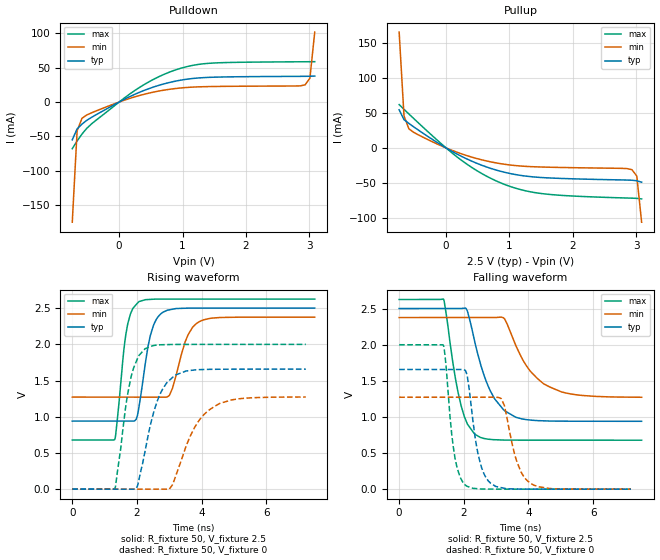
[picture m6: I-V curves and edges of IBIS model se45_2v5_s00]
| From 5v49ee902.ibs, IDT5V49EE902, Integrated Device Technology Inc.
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[Model]   se45_2v5_s00
Model_type   Output
Polarity   Non-Inverting
|   typ   min   max
C_comp   2pF   1.5pF   2.5pF
Vmeas = 1.25V
Rref = 50
Cref = 0
Vref = 1.25V
|   typ   min   max
[Voltage range]   2.5V   2.375V   2.625V
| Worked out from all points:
|   slope of the pulldown table from 0 to 0.375 V, typ, clamps not added: 23.2 ohm
|   slope of the pullup table from 0 to 0.375 V, typ, clamps not added: 21 ohm
|   rising waveform, R_fixture 50, V_fixture 2.5: 20-80 % time 355ps typ, 450ps min, 276ps max; typ from 0.939 V to 2.5 V
|   falling waveform, R_fixture 50, V_fixture 2.5: 20-80 % time 687ps typ, 919ps min, 460ps max; typ from 2.5 V to 0.939 V
|   rising waveform, R_fixture 50, V_fixture 0: 20-80 % time 568ps typ, 790ps min, 399ps max; typ from 0 V to 1.66 V
|   falling waveform, R_fixture 50, V_fixture 0: 20-80 % time 345ps typ, 432ps min, 272ps max; typ from 1.66 V to 0 V
[Pulldown]
|Voltage   I (typ)   I (min)   I (max)
|Note, modeling breaks down at 250mA and above.  This is well beyond the functional   |
|operating range of the device.  Should this scenario occur, catastrophic failure and   |
|possible damage to the device and/or board is of higher concern than the I-V curve   |
|behavior.  The IBIS checker will flag currents in excess of 10A with warnings.  Lines   |
|with currents in excess of 0.35 A have been commented out.  The points still remain|
|available to the user if the user desires to use them.   |
|-2.50000e+00   -4.54709e+01   -3.63694e+01   -6.07959e+01
|-2.42347e+00   -4.32502e+01   -3.46594e+01   -5.77053e+01
|-2.34694e+00   -4.10314e+01   -3.29511e+01   -5.46170e+01
|-2.27041e+00   -3.88148e+01   -3.12446e+01   -5.15313e+01
|-2.19388e+00   -3.66007e+01   -2.95401e+01   -4.84486e+01
|-2.11735e+00   -3.43893e+01   -2.78380e+01   -4.53691e+01
|-2.04082e+00   -3.21809e+01   -2.61384e+01   -4.22934e+01
|-1.96429e+00   -2.99761e+01   -2.44418e+01   -3.92219e+01
|-1.88776e+00   -2.77753e+01   -2.27484e+01   -3.61555e+01
|-1.81122e+00   -2.55791e+01   -2.10589e+01   -3.30948e+01
|-1.73469e+00   -2.33884e+01   -1.93737e+01   -3.00411e+01
|-1.65816e+00   -2.12042e+01   -1.76937e+01   -2.69958e+01
|-1.58163e+00   -1.90279e+01   -1.60198e+01   -2.39607e+01
|-1.50510e+00   -1.68611e+01   -1.43533e+01   -2.09385e+01
|-1.42857e+00   -1.47065e+01   -1.26960e+01   -1.79331e+01
|-1.35204e+00   -1.25675e+01   -1.10500e+01   -1.49501e+01
|-1.27551e+00   -1.04495e+01   -9.41889e+00   -1.19989e+01
|-1.19898e+00   -8.36102e+00   -7.80755e+00   -9.09553e+00
|-1.12245e+00   -6.31683e+00   -6.22400e+00   -6.27207e+00
|-1.04592e+00   -4.34540e+00   -4.68188e+00   -3.60463e+00
|-9.69388e-01   -2.51112e+00   -3.20700e+00   -1.33260e+00
|-8.92857e-01   -9.89892e-01   -1.85502e+00   -2.01598e-01
|-8.16327e-01   -1.92135e-01   -7.61074e-01   -8.24374e-02
-739.8mV  -54.82mA   -174.4mA   -67.73mA
-663.3mV  -39mA      -41.68mA   -56.5mA
-586.7mV  -31.96mA   -23.62mA   -46.47mA
-433.7mV  -22.15mA   -15.6mA    -31.55mA
255.1mV   11.54mA    7.746mA    17.23mA
637.8mV   24.55mA    16.14mA    37.26mA
943.9mV   31.29mA    20.16mA    48.22mA
1.173V    34.28mA    21.72mA    53.44mA
1.48V     36mA       22.52mA    56.56mA
2.934V    37.31mA    24.91mA    58.47mA
3.01V     37.39mA    34.58mA    58.51mA
3.087V    37.69mA    101.5mA    58.57mA
| 3.16327e+00   3.94370e-02   3.90716e-01   5.87161e-02
| 3.23980e+00   5.34569e-02   9.26332e-01   5.92247e-02
| 3.31633e+00   1.87777e-01   1.58664e+00   6.05142e-02
| 3.39286e+00   7.03900e-01   2.30650e+00   6.31621e-02
| 3.46939e+00   1.49296e+00   3.05902e+00   8.17834e-02
| 3.54592e+00   2.39302e+00   3.83167e+00   3.62573e-01
| 3.62245e+00   3.34512e+00   4.61786e+00   1.23067e+00
| 3.69898e+00   4.32630e+00   5.41369e+00   2.35283e+00
| 3.77551e+00   5.32579e+00   6.21672e+00   3.56536e+00
| 3.85204e+00   6.33779e+00   7.02533e+00   4.82080e+00
| 3.92857e+00   7.35883e+00   7.83838e+00   6.10084e+00
| 4.00510e+00   8.38670e+00   8.65504e+00   7.39669e+00
| 4.08163e+00   9.41993e+00   9.47469e+00   8.70352e+00
| 4.15816e+00   1.04574e+01   1.02969e+01   1.00184e+01
| 4.23469e+00   1.14984e+01   1.11212e+01   1.13394e+01
| 4.31122e+00   1.25424e+01   1.19474e+01   1.26653e+01
| 4.38776e+00   1.35888e+01   1.27751e+01   1.39952e+01
| 4.46429e+00   1.46373e+01   1.36044e+01   1.53282e+01
| 4.54082e+00   1.56877e+01   1.44348e+01   1.66640e+01
| 4.61735e+00   1.67397e+01   1.52665e+01   1.80021e+01
| 4.69388e+00   1.77932e+01   1.60991e+01   1.93422e+01
| 4.77041e+00   1.88479e+01   1.69326e+01   2.06841e+01
| 4.84694e+00   1.99037e+01   1.77670e+01   2.20275e+01
| 4.92347e+00   2.09606e+01   1.86021e+01   2.33723e+01
| 5.00000e+00   2.20184e+01   1.94379e+01   2.47183e+01
[Pullup]
|Voltage   I (typ)   I (min)   I (max)
|Note, modeling breaks down at 250mA and above.  This is well beyond the functional   |
|operating range of the device.  Should this scenario occur, catastrophic failure and   |
|possible damage to the device and/or board is of higher concern than the I-V curve   |
|behavior.  The IBIS checker will flag currents in excess of 10A with warnings.  Lines   |
|with currents in excess of 0.35 A have been commented out.  The points still remain|
|available to the user if the user desires to use them.   |
|-2.50000e+00   2.19765e+01   1.80472e+01   2.68517e+01
|-2.42347e+00   2.09191e+01   1.72127e+01   2.55048e+01
|-2.34694e+00   1.98626e+01   1.63791e+01   2.41589e+01
|-2.27041e+00   1.88071e+01   1.55463e+01   2.28141e+01
|-2.19388e+00   1.77528e+01   1.47145e+01   2.14705e+01
|-2.11735e+00   1.66997e+01   1.38838e+01   2.01283e+01
|-2.04082e+00   1.56480e+01   1.30543e+01   1.87877e+01
|-1.96429e+00   1.45980e+01   1.22261e+01   1.74489e+01
|-1.88776e+00   1.35497e+01   1.13995e+01   1.61122e+01
|-1.81122e+00   1.25036e+01   1.05747e+01   1.47780e+01
|-1.73469e+00   1.14600e+01   9.75186e+00   1.34466e+01
|-1.65816e+00   1.04193e+01   8.93142e+00   1.21187e+01
|-1.58163e+00   9.38215e+00   8.11380e+00   1.07950e+01
|-1.50510e+00   8.34928e+00   7.29955e+00   9.47668e+00
|-1.42857e+00   7.32178e+00   6.48942e+00   8.16516e+00
|-1.35204e+00   6.30119e+00   5.68442e+00   6.86272e+00
|-1.27551e+00   5.28973e+00   4.88602e+00   5.57292e+00
|-1.19898e+00   4.29091e+00   4.09630e+00   4.30185e+00
|-1.12245e+00   3.31066e+00   3.31857e+00   3.06117e+00
|-1.04592e+00   2.36002e+00   2.55827e+00   1.87712e+00
|-9.69388e-01   1.46263e+00   1.82537e+00   8.26238e-01
|-8.92857e-01   6.79721e-01   1.14025e+00   1.77022e-01
|-8.16327e-01   1.78304e-01   5.50947e-01   7.20287e-02
-739.8mV  54.64mA    166.3mA    62.19mA
-663.3mV  40.61mA    45.96mA    55.4mA
-586.7mV  35.13mA    27.42mA    48.78mA
-204.1mV  11.53mA    8.292mA    16.47mA
255.1mV   -12.67mA   -8.857mA   -18.54mA
561.2mV   -24.84mA   -17.08mA   -36.7mA
943.9mV   -35.45mA   -23.78mA   -53.18mA
1.25V     -40.42mA   -26.48mA   -61.53mA
1.556V    -42.81mA   -27.59mA   -66.09mA
2.934V    -46.44mA   -31.28mA   -72.19mA
3.01V     -47.21mA   -40.39mA   -72.48mA
3.087V    -49.28mA   -106.7mA   -73.28mA
| 3.16327e+00   -5.35776e-02   -4.94236e-01   -7.58575e-02
| 3.23980e+00   -6.85824e-02   -1.43626e+00   -8.09811e-02
| 3.31633e+00   -2.12479e-01   -2.71822e+00   -8.81300e-02
| 3.39286e+00   -1.02359e+00   -4.15794e+00   -9.69442e-02
| 3.46939e+00   -2.55073e+00   -5.67974e+00   -1.18777e-01
| 3.54592e+00   -4.38708e+00   -7.25021e+00   -4.69271e-01
| 3.62245e+00   -6.35927e+00   -8.85247e+00   -2.14689e+00
| 3.69898e+00   -8.40369e+00   -1.04769e+01   -4.62063e+00
| 3.77551e+00   -1.04921e+01   -1.21177e+01   -7.36117e+00
| 3.85204e+00   -1.26099e+01   -1.37710e+01   -1.02197e+01
| 3.92857e+00   -1.47486e+01   -1.54342e+01   -1.31429e+01
| 4.00510e+00   -1.69029e+01   -1.71053e+01   -1.61066e+01
| 4.08163e+00   -1.90692e+01   -1.87829e+01   -1.90980e+01
| 4.15816e+00   -2.12452e+01   -2.04660e+01   -2.21093e+01
| 4.23469e+00   -2.34289e+01   -2.21537e+01   -2.51357e+01
| 4.31122e+00   -2.56192e+01   -2.38455e+01   -2.81738e+01
| 4.38776e+00   -2.78148e+01   -2.55407e+01   -3.12215e+01
| 4.46429e+00   -3.00151e+01   -2.72389e+01   -3.42769e+01
| 4.54082e+00   -3.22195e+01   -2.89399e+01   -3.73388e+01
| 4.61735e+00   -3.44273e+01   -3.06432e+01   -4.04061e+01
| 4.69388e+00   -3.66382e+01   -3.23486e+01   -4.34782e+01
| 4.77041e+00   -3.88519e+01   -3.40560e+01   -4.65543e+01
| 4.84694e+00   -4.10679e+01   -3.57652e+01   -4.96340e+01
| 4.92347e+00   -4.32862e+01   -3.74759e+01   -5.27168e+01
| 5.00000e+00   -4.55064e+01   -3.91880e+01   -5.58024e+01
[Ramp]
|   typ   min   max
dV/dt_r   0.936/0.355n   0.663/0.45n   1.168/0.276n
dV/dt_f   0.94/0.687n  0.665/0.92n   1.172/0.46n
R_load =   50
[Rising Waveform]
R_fixture = 50
V_fixture = 2.5   |Vcc_typ
V_fixture_min = 2.375 |Vcc_min
V_fixture_max = 2.625 |Vcc_max
C_fixture = 0.0p
| Time   typ   min   max
0s        939.3mV    1.271V     677.7mV
1.312ns   939.3mV    1.271V     683.9mV
1.69ns    939.3mV    1.271V     2.224V
2.065ns   1.143V     1.271V     2.591V
2.411ns   2.115V     1.271V     2.621V
2.812ns   2.445V     1.27V      2.625V
3.003ns   2.476V     1.294V     2.625V
3.486ns   2.498V     2.028V     2.625V
3.93ns    2.5V       2.313V     2.625V
7.5ns     2.5V       2.375V     2.625V
[Falling Waveform]
R_fixture = 50
V_fixture = 2.5   |Vcc_typ
V_fixture_min = 2.375 |Vcc_min
V_fixture_max = 2.625 |Vcc_max
C_fixture = 0.0p
| Time   typ   min   max
0s        2.5V       2.375V     2.625V
1.373ns   2.5V       2.375V     2.628V
1.918ns   2.501V     2.375V     1.152V
2.112ns   2.464V     2.375V     900mV
2.5ns     1.755V     2.375V     718mV
3.224ns   1.102V     2.372V     679.8mV
3.612ns   994.7mV    1.984V     678.2mV
4.1ns     954.4mV    1.612V     678mV
5ns       941mV      1.349V     677.9mV
7.5ns     939.4mV    1.272V     677.8mV
[Rising Waveform]
R_fixture = 50
V_fixture = 0
C_fixture = 0.0p
| Time   typ   min   max
0s        96.64nV    102.5nV    85.59nV
1.314ns   79.59nV    102.5nV    1.765mV
1.818ns   -71.84uV   130.8nV    1.549V
2.015ns   40.51mV    84.33nV    1.801V
2.253ns   529.4mV    -327nV     1.94V
2.671ns   1.265V     84.19uV    1.992V
3.215ns   1.58V      201.3mV    1.998V
3.788ns   1.646V     854.6mV    1.999V
4.414ns   1.655V     1.146V     1.999V
7.224ns   1.657V     1.272V     1.999V
[Falling Waveform]
R_fixture = 50
V_fixture = 0
C_fixture = 0.0p
| Time   typ   min   max
0s        1.657V     1.272V     1.999V
1.366ns   1.657V     1.272V     1.993V
1.729ns   1.657V     1.272V     424.6mV
2.081ns   1.61V      1.272V     44.97mV
2.437ns   493.2mV    1.272V     5.062mV
2.838ns   78.74mV    1.272V     618.9uV
3.157ns   21.01mV    1.253V     274.9uV
3.65ns    1.105mV    370.1mV    181.4uV
4.067ns   489uV      81.99mV    145.4uV
7.169ns   116.3uV    256.9uV    57.2uV
